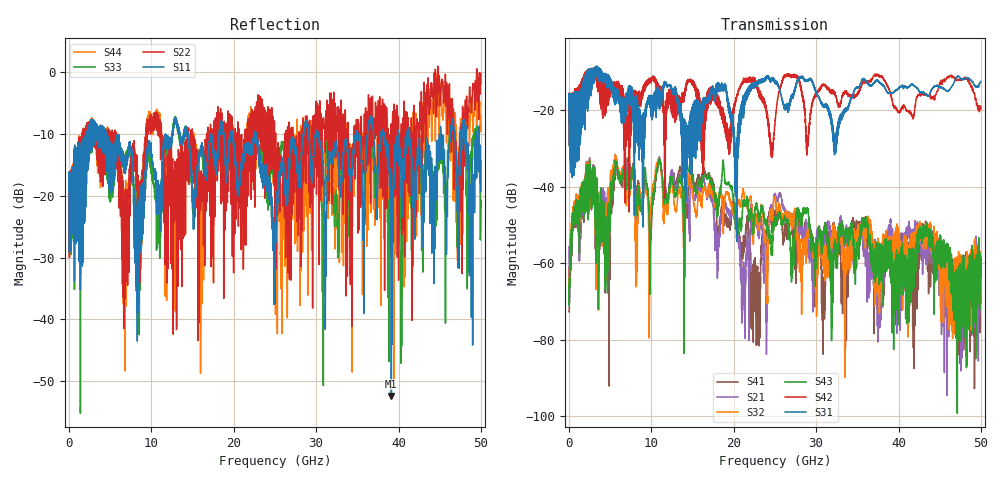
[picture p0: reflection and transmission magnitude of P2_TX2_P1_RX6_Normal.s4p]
!Keysight Technologies,N5225B,MY57041031,A.13.20.10
!Date: Friday, May 31, 2019 11:23:12
!Correction: S11(Full 4 Port(1,2,3,4))
!S12(Full 4 Port(1,2,3,4))
!S13(Full 4 Port(1,2,3,4))
!S14(Full 4 Port(1,2,3,4))
!S21(Full 4 Port(1,2,3,4))
!S22(Full 4 Port(1,2,3,4))
!S23(Full 4 Port(1,2,3,4))
!S24(Full 4 Port(1,2,3,4))
!S31(Full 4 Port(1,2,3,4))
!S32(Full 4 Port(1,2,3,4))
!S33(Full 4 Port(1,2,3,4))
!S34(Full 4 Port(1,2,3,4))
!S41(Full 4 Port(1,2,3,4))
!S42(Full 4 Port(1,2,3,4))
!S43(Full 4 Port(1,2,3,4))
!S44(Full 4 Port(1,2,3,4))
!S4P File: Measurements: <S11,S12,S13,S14>,
!<S21,S22,S23,S24>,
!<S31,S32,S33,S34>,
!<S41,S42,S43,S44>:
# Hz S  dB  R 50.0
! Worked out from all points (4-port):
!   5000 points, 10 MHz to 50 GHz, reference 50 ohm
!   strongest paths, dB at 10 MHz, 12.51 GHz, 25.01 GHz, 37.51 GHz, 50 GHz:
!     S31: -19.3, -14.8, -13.0, -12.4, -12.6
!     S42: -19.5, -15.6, -22.9, -10.8, -19.3
!     S43: -67.8, -38.2, -49.3, -60.6, -62.2
!     S32: -63.6, -39.3, -42.6, -60.2, -59.3
!     S21: -55.7, -36.3, -41.7, -75.0, -63.9
!     S41: -72.7, -36.4, -47.5, -61.7, -70.5
!   lowest |S11| = -52.5 dB at 39.13 GHz (marker M1), VSWR 1.00, Z = 50.2 + j0.123 ohm
!   |S11| at or under -10 dB: 4.481 GHz to 11.72 GHz (7.238 GHz wide, 89.4 % of centre); 22.73 GHz to 28.43 GHz (5.702 GHz wide, 22.3 % of centre); 30.26 GHz to 34.82 GHz (4.558 GHz wide, 14 % of centre)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
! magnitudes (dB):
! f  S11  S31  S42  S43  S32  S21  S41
! 10 MHz  -19.1  -19.3  -19.5  -67.8  -63.6  -55.7  -72.7
! 2.3 GHz  -15.8  -19.4  -12.4  -39.7  -39.7  -39.0  -39.2
! 7.06 GHz  -14.0  -15.8  -24.0  -36.5  -38.2  -34.6  -32.9
! 21.15 GHz  -13.8  -16.2  -13.0  -44.9  -41.0  -70.8  -54.5
! 25.07 GHz  -25.5  -12.8  -21.7  -48.4  -44.3  -42.4  -46.8
! 39.13 GHz  -52.5  -15.6  -16.8  -65.3  -59.5  -52.4  -56.3
! 50 GHz  -14.3  -12.6  -19.3  -62.2  -59.3  -63.9  -70.5
